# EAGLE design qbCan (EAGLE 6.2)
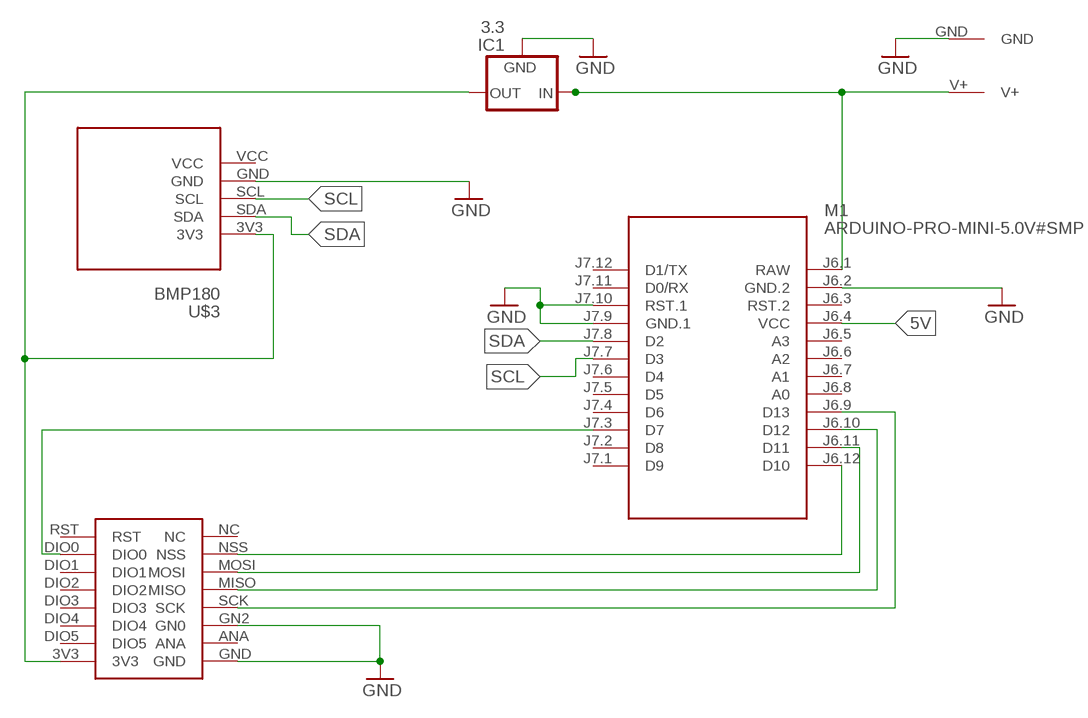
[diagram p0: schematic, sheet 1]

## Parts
IC1  3.3  LD1117  [TO220L1]
M1  ARDUINO-PRO-MINI-5.0V#SMP  [ARDUINO-PRO-MINI#SMP]
U$2  BATTERY  [BATTERY]
U$3  BMP180  [BMP180]
U$5  RFM69-TH  [RFM69-TH]

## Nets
5V: M1.J6.4(VCC)
GND: IC1.1(GND) M1.J6.2(GND.2) M1.J7.9(GND.1) M1.J7.10(RST.1) U$2.GND U$3.GND U$5.GN2(GN0) U$5.GND
N$1: M1.J7.3(D7) U$5.DIO0
N$2: IC1.3(IN) M1.J6.1(RAW) U$2.V+
N$3: IC1.2(OUT) U$3.3V3 U$5.3V3
N$6: M1.J6.12(D10) U$5.NSS
N$7: M1.J6.11(D11) U$5.MOSI
N$8: M1.J6.9(D13) U$5.SCK
N$10: M1.J6.10(D12) U$5.MISO
SCL: M1.J7.7(D3) U$3.SCL
SDA: M1.J7.8(D2) U$3.SDA
Unconnected: M1.J6.3(RST.2) M1.J6.5(A3) M1.J6.6(A2) M1.J6.7(A1) M1.J6.8(A0) M1.J7.1(D9) M1.J7.2(D8) M1.J7.4(D6) M1.J7.5(D5) M1.J7.6(D4) M1.J7.11(D0/RX) M1.J7.12(D1/TX) U$3.VCC U$5.ANA U$5.DIO1 U$5.DIO2 U$5.DIO3 U$5.DIO4 U$5.DIO5 U$5.NC U$5.RST

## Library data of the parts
IC1 = qbCan:LD1117: VOLTAGE REGULATOR
M1 = qbCan:ARDUINO-PRO-MINI-*#SMP: Arduino Pro Mini with 2 connectors only
U$2 = qbCan:BATTERY
U$3 = qbCan:BMP180
U$5 = qbCan:RFM69-TH

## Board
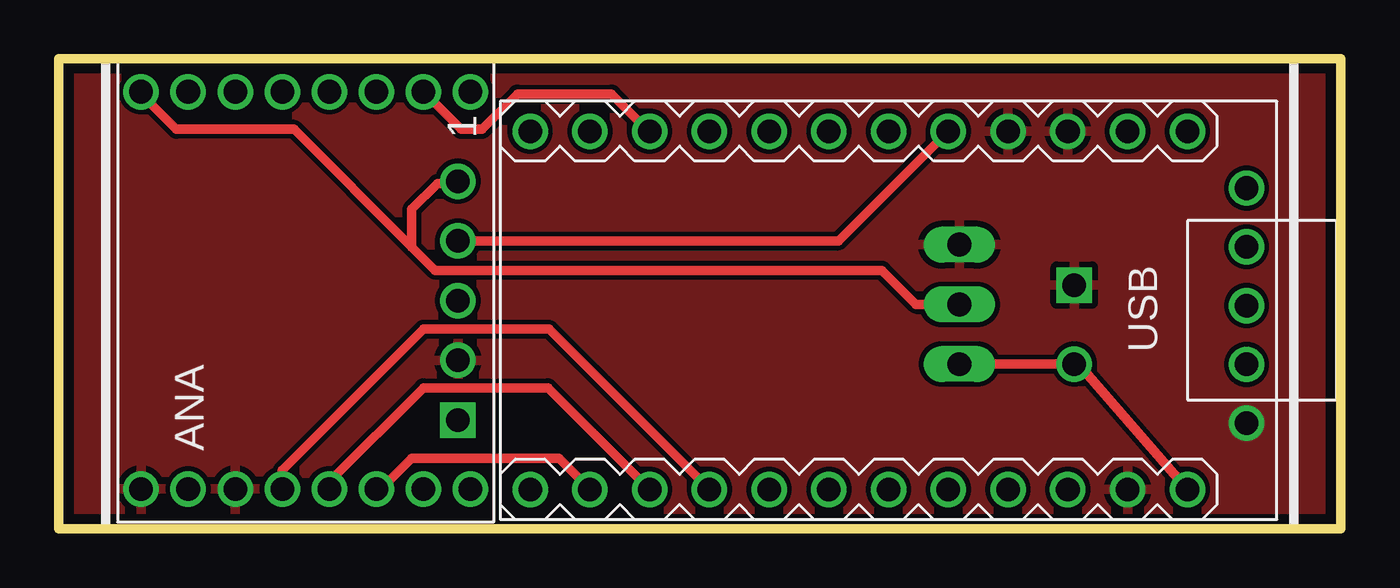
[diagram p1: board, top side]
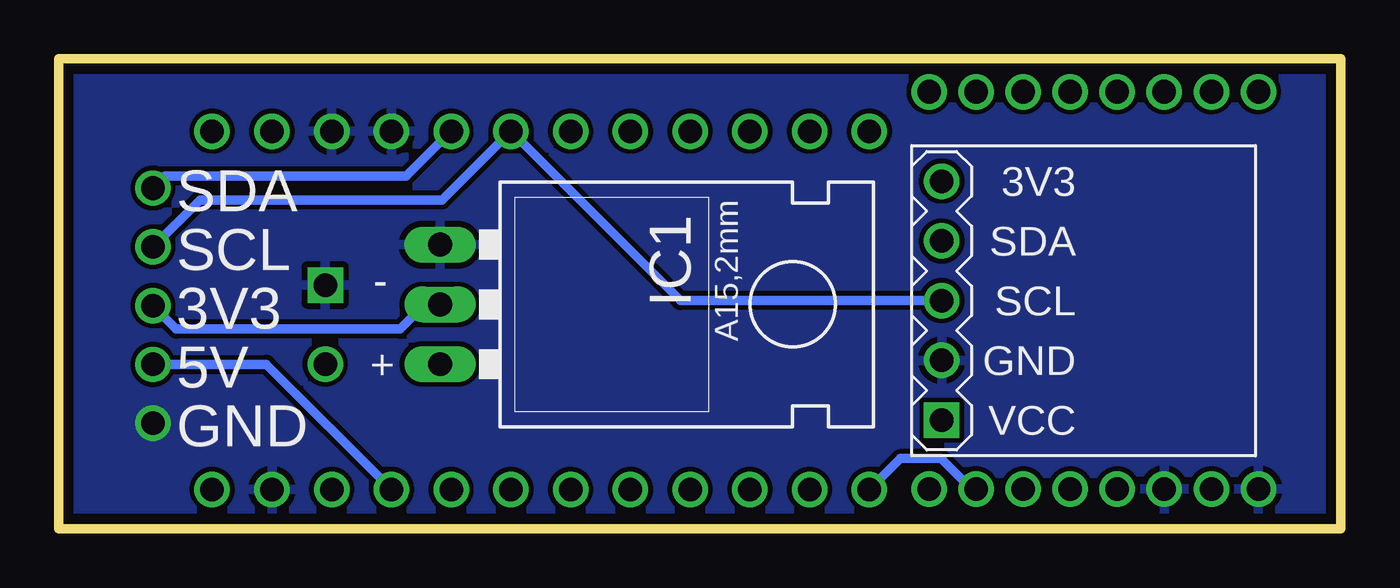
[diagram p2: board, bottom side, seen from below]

Size 54.5 x 20 mm. Coordinates in mm from the lower left corner, seen from the top.
Outline: 0,0 54.5,0 54.5,20 0,20 0,0
Copper layers (1*16): Top 0.035mm / dielectric 1.5mm / Bottom 0.035mm
Design rules: minimum track width 10mil, minimum drill 24mil, track to track 8mil, track to pad 8mil, pad to pad 8mil, via to via 8mil, smd to smd 8mil, copper to edge 17mil, drill to drill 8mil, minimum pad ring 10mil, minimum via ring 8mil, stop-mask expansion 4mil, vias tented up to drill 0mil, thermal gap 10mil

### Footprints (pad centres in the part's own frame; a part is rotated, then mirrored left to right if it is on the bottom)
TO220L1 = drill 1.016 long: 1 -2.54,-3.81; 2 0,-3.81; 3 2.54,-3.81
ARDUINO-PRO-MINI#SMP = drill 1: J6.1 -12.7,7.62; J6.2 -10.16,7.62; J6.3 -7.62,7.62; J6.4 -5.08,7.62; J6.5 -2.54,7.62; J6.6 0,7.62; J6.7 2.54,7.62; J6.8 5.08,7.62; J6.9 7.62,7.62; J6.10 10.16,7.62; J6.11 12.7,7.62; J6.12 15.24,7.62; J7.1 15.24,-7.62; J7.2 12.7,-7.62; J7.3 10.16,-7.62; J7.4 7.62,-7.62; J7.5 5.08,-7.62; J7.6 2.54,-7.62; J7.7 0,-7.62; J7.8 -2.54,-7.62; J7.9 -5.08,-7.62; J7.10 -7.62,-7.62; J7.11 -10.16,-7.62; J7.12 -12.7,-7.62
BATTERY = drill 1 square: GND 0,3.365 | drill 1: V+ 0,0
BMP180 = drill 1: 3V3 5.715,-5.08; GND 5.715,2.54; SCL 5.715,0; SDA 5.715,-2.54 | drill 1 square: VCC 5.715,5.08
RFM69-TH = drill 1: 3V3 1.4,1; ANA 18.3,3; DIO0 1.4,13; DIO1 1.4,11; DIO2 1.4,9; DIO3 1.4,7; DIO4 1.4,5; DIO5 1.4,3; GN2 18.3,5; GND 18.3,1; MISO 18.3,9; MOSI 18.3,11; NC 18.3,15; NSS 18.3,13; RST 1.4,15; SCK 18.3,7

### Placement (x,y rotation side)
IC1  34.48,9.55 270 bottom
M1  35.28,9.3 180 top
U$2  43.17,7.01 0 bottom
U$3  11.25,9.71 180 bottom
U$5  2.5,20 270 top

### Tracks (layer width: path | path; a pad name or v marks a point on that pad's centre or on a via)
5V  (via drill 1)
  Bottom 0.406: v50.5,7 45.68,7 M1.J6.4
GND  (via drill 1)
  other vias: 50.5,4.5
  pour Bottom: 0,0 54.5,0 54.5,20 0,20
  pour Top: 0,0 54.5,0 54.5,20 0,20
N$1
  Top 0.406: U$5.DIO0 17.1,17 18,17 19.5,18.5 23.5,18.5 25.08,16.92 M1.J7.3
N$2
  Top 0.406: IC1.3 U$2.V+ 43.35,7.01 M1.J6.1
N$3  (via drill 1)
  Top 0.406: IC1.2 36.45,9.55 35,11 16,11 15,12 | U$3.3V3 16.88,14.7 16.1,14.7 15,13.6 15,12 | 15,12 10,17 5,17 3.5,18.5 U$5.3V3
  Bottom 0.406: IC1.2 38.95,9.55 40,8.5 49.5,8.5 v50.5,9.5
N$6
  Bottom 0.406: U$5.NSS 15.7,1.7 17,3 18.72,3 M1.J6.12
N$7
  Top 0.406: U$5.MOSI 13.7,1.7 15,3 21.26,3 M1.J6.11
N$8
  Top 0.406: U$5.SCK 9.5,2.5 15.5,8.5 20.84,8.5 M1.J6.9
N$10
  Top 0.406: U$5.MISO 11.5,2 15.5,6 20.8,6 M1.J6.10
SCL  (via drill 1)
  Bottom 0.406: U$3.SCL 28.07,9.71 M1.J7.7 38.2,14 48.5,14 v50.5,12
SDA  (via drill 1)
  Top 0.406: U$3.SDA 33.15,12.25 M1.J7.8
  Bottom 0.406: M1.J7.8 39.74,15 50,15 v50.5,14.5

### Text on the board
bPlace: SDA | SCL | 3V3 | 5V | GND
